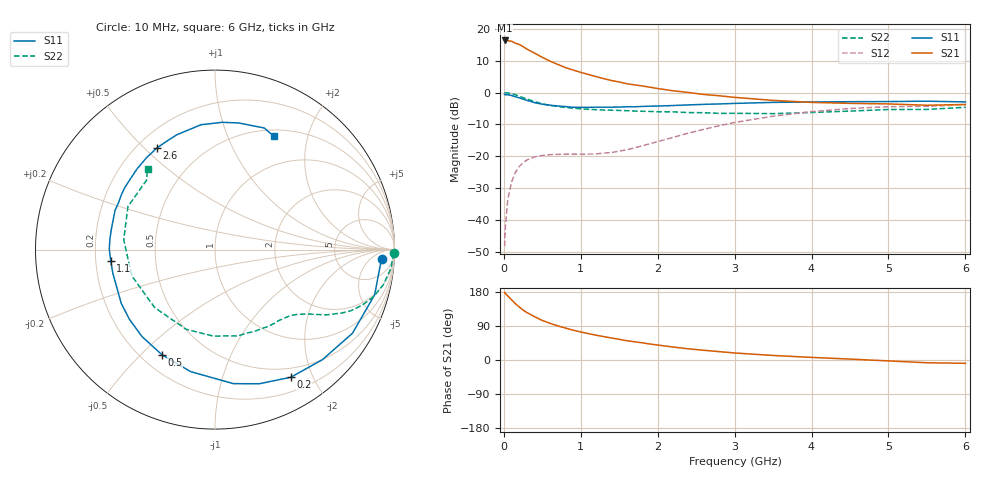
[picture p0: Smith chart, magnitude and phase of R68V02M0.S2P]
! SIEMENS Small Signal Semiconductors
! BFR193
! Si NPN RF Bipolar Junction Transistor in SOT23
! VCE = 8 V  IC = 2 mA
! Common Emitter S-Parameters:  May  1996
# GHz  S  MA  R  50
!  f  S11  S21  S12  S22
! GHz  MAG  ANG  MAG  ANG  MAG  ANG  MAG  ANG
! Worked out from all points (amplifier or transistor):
!   36 points, 10 MHz to 6 GHz, reference 50 ohm
!   highest |S21| = 16.3 dB at 10 MHz (marker M1)
!   |S21| within 3 dB of that: start of sweep to 322.9 MHz
!   unconditionally stable (mu >= 1): 1.175 GHz to 2.066 GHz
!   at 250 MHz: K = 0.23, MSG = 18.2 dB, |S12| = -22.0 dB
!   at 1.4 GHz: K = 1.12, MAG = 9.2 dB, |S12| = -18.8 dB
!   at 6 GHz: K = 0.99, MSG = 0.1 dB, |S12| = -3.9 dB
!   S11 on the Smith chart (normalised r, x): 10 MHz: 17, -13; 200 MHz: 0.38, -1.69; 500 MHz: 0.28, -0.58; 1.1 GHz: 0.26, -0.05; 2.6 GHz: 0.28, +0.55; 6 GHz: 0.58, +1.48
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0.01  0.9292 -3.2  6.545 178.2  0.0039 87.5  0.9973 -1.2
0.02  0.9237 -6.4  6.41 175.6  0.008 85.5  0.9916 -2.4
0.05  0.9244 -15.8  6.504 169.3  0.0206 80.1  0.9863 -6.0
0.1  0.8966 -31.3  6.36 159.0  0.0393 73.4  0.9589 -11.7
0.15  0.8569 -45.7  5.935 148.7  0.0559 65.2  0.9214 -16.6
0.2  0.8272 -59.3  5.661 139.9  0.0692 58.8  0.8762 -20.7
0.25  0.787 -71.8  5.236 131.8  0.0791 52.4  0.8291 -24.3
0.3  0.7537 -82.2  4.79 125.2  0.0875 48.4  0.7891 -26.6
0.4  0.6933 -101.3  4.143 114.1  0.0981 41.6  0.7205 -30.3
0.5  0.6561 -116.8  3.556 104.4  0.103 37.1  0.6648 -32.9
0.6  0.6326 -130.0  3.105 96.8  0.1061 34.5  0.6288 -34.8
0.7  0.615 -140.8  2.757 90.1  0.1072 33.1  0.6049 -36.5
0.9  0.5863 -158.9  2.25 78.8  0.1081 33.9  0.5679 -39.9
1.1  0.5844 -173.8  1.913 69.6  0.1084 38.1  0.5452 -44.1
1.3  0.5886 174.2  1.647 61.7  0.1123 44.1  0.5309 -48.4
1.6  0.5982 158.6  1.371 50.8  0.1268 54.1  0.5188 -56.1
2.2  0.6252 134.0  1.064 34.2  0.1978 64.4  0.4977 -75.2
2.6  0.652 119.8  0.932 25.6  0.2647 63.0  0.482 -91.2
3.5  0.7001 96.4  0.752 12.0  0.4252 48.4  0.4663 -136.2
4.5  0.7177 79.5  0.676 2.4  0.5607 27.4  0.5115 173.8
5.5  0.7309 68.0  0.631 -7.3  0.6082 7.8  0.543 134.7
6  0.712 62.7  0.649 -8.7  0.6411 2.5  0.5857 129.9
